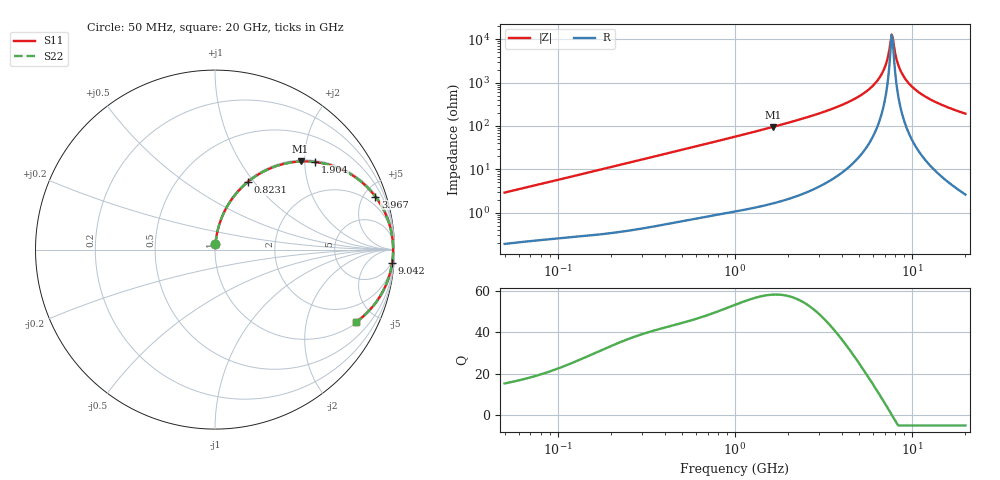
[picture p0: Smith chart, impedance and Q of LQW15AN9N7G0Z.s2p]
!Murata Part Number: LQW15AN9N7G0Z
!These Parameters are Measured in Series Mode Connection
!  o--[Z]--o
!Port1  Port2
!  o-------o
!Freq. Start=50[MHz] Stop=20[GHz], 401[Steps]
# Hz S RI R 50
!Freq.(Hz) S11(Real) S11(Imag) S21(Real) S21(Imag) S12(Real) S12(Imag) S22(Real) S22(Imag)
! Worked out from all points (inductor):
!   401 points, 50 MHz to 20 GHz, reference 50 ohm
!   read as one part in series: L = 9.2 nH near 51.52 MHz
!   highest Q = 58.1 at 1.639 GHz (marker M1), where L = 9.25 nH
!   self-resonance near 7.668 GHz
!   S11 on the Smith chart (normalised r, x): 50 MHz: 1.00, +0.06; 823.1 MHz: 1.02, +0.93; 1.904 GHz: 1.04, +2.25; 3.967 GHz: 1.16, +5.98; 9.042 GHz: 4, -26; 20 GHz: 1.05, -3.85
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5e7  0.00275 0.029  0.9973 -0.029  0.9973 -0.029  0.00275 0.029
1.364002e8  0.0088 0.0768  0.9912 -0.0768  0.9912 -0.0768  0.0088 0.0768
3.721004e8  0.0467 0.1993  0.9533 -0.1993  0.9533 -0.1993  0.0467 0.1993
8.230629e8  0.1824 0.3764  0.8176 -0.3764  0.8176 -0.3764  0.1824 0.3764
1e9  0.2471 0.422  0.7529 -0.422  0.7529 -0.422  0.2471 0.422
1.639343e9  0.4765 0.4909  0.5235 -0.4909  0.5235 -0.4909  0.4765 0.4909
1.904239e9  0.5578 0.4881  0.4422 -0.4881  0.4422 -0.4881  0.5578 0.4881
2.728004e9  0.7453 0.4261  0.2547 -0.4261  0.2547 -0.4261  0.7453 0.4261
3.967106e9  0.8931 0.2957  0.1069 -0.2957  0.1069 -0.2957  0.8931 0.2957
5.194772e9  0.9581 0.1799  0.0419 -0.1799  0.0419 -0.1799  0.9581 0.1799
6.217679e9  0.9824 0.0984  0.0176 -0.0984  0.0176 -0.0984  0.9824 0.0984
6.701223e9  0.9882 0.064  0.0118 -0.064  0.0118 -0.064  0.9882 0.064
7.009217e9  0.9905 0.0433  0.00948 -0.0433  0.00948 -0.0433  0.9905 0.0433
7.222371e9  0.9916 0.0295  0.00843 -0.0295  0.00843 -0.0295  0.9916 0.0295
7.442007e9  0.9922 0.0156  0.00777 -0.0156  0.00777 -0.0156  0.9922 0.0156
7.554318e9  0.9924 0.0087  0.00758 -0.0087  0.00758 -0.0087  0.9924 0.0087
7.784049e9  0.9925 -0.00514  0.0075 0.00514  0.0075 0.00514  0.9925 -0.00514
8.389408e9  0.991 -0.0397  0.00899 0.0397  0.00899 0.0397  0.991 -0.0397
9.041845e9  0.9871 -0.0743  0.0129 0.0743  0.0129 0.0743  0.9871 -0.0743
1.019291e10  0.9756 -0.1292  0.0244 0.1292  0.0244 0.1292  0.9756 -0.1292
1.201863e10  0.9492 -0.2035  0.0508 0.2035  0.0508 0.2035  0.9492 -0.2035
2e10  0.7845 -0.4044  0.2155 0.4044  0.2155 0.4044  0.7845 -0.4044
